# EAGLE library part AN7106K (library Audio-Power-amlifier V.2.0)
Single Chip Stereo Pre-amplifier/ Power Amplifier
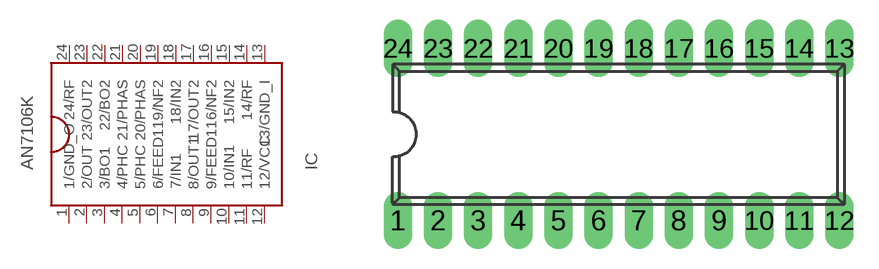
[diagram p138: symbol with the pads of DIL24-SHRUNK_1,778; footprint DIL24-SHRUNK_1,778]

Designator prefix IC

## AN7106K  [DIL24-SHRUNK_1,778]
1  1/GND_O  pwr
2  2/OUT  out
3  3/BO1
4  4/PHC
5  5/PHC
6  6/FEED1  in
7  7/IN1  in
8  8/OUT1  out
9  9/FEED1  in
10  10/IN1  in
11  11/RF
12  12/VCC  pwr
13  13/GND_I  pwr
14  14/RF
15  15/IN2  in
16  16/NF2  in
17  17/OUT2  out
18  18/IN2  in
19  19/NF2  in
20  20/PHAS
21  21/PHAS
22  22/BO2
23  23/OUT2  out
24  24/RF

## Footprint DIL24-SHRUNK_1,778 (pad centres in mm)
24-Lead Shrunk DIL Plastic Package
drill 0.6 pad 1.27 long: 1 -10.667,-3.812; 2 -8.889,-3.811; 3 -7.111,-3.81; 4 -5.333,-3.81; 5 -3.555,-3.811; 6 -1.777,-3.811; 7 0.001,-3.811; 8 1.778,-3.811; 9 3.557,-3.811; 10 5.335,-3.811; 11 7.113,-3.811; 12 8.891,-3.811; 13 8.892,3.81; 14 7.113,3.81; 15 5.335,3.81; 16 3.557,3.81; 17 1.779,3.81; 18 0.001,3.81; 19 -1.777,3.81; 20 -3.556,3.81; 21 -5.333,3.809; 22 -7.112,3.81; 23 -8.889,3.81; 24 -10.667,3.81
